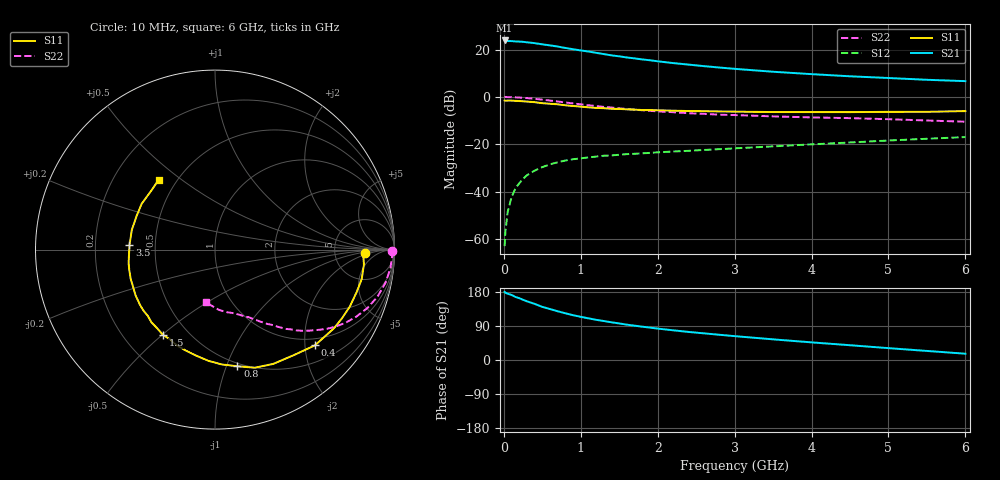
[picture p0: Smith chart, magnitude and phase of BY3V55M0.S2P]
! SIEMENS Small Signal Semiconductors
! BFY420
! Si NPN RF SIEGET Grounded Emitter Transistor in MICRO-X
! VCE = 3.5 V  IC = 5 mA
! Common Emitter S-Parameters:  October  1996
# GHz  S  MA  R  50
!  f  S11  S21  S12  S22
! GHz  MAG  ANG  MAG  ANG  MAG  ANG  MAG  ANG
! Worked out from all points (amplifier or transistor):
!   36 points, 10 MHz to 6 GHz, reference 50 ohm
!   highest |S21| = 23.8 dB at 10 MHz (marker M1)
!   |S21| within 3 dB of that: start of sweep to 771.4 MHz
!   unconditionally stable (mu >= 1): 3.175 GHz to end of sweep
!   at 250 MHz: K = 0.15, MSG = 28.9 dB, |S12| = -34.7 dB
!   at 1.4 GHz: K = 0.53, MSG = 21.1 dB, |S12| = -24.7 dB
!   at 6 GHz: K = 1.13, MAG = 9.6 dB, |S12| = -17.0 dB
!   S11 on the Smith chart (normalised r, x): 10 MHz: 11, -1; 400 MHz: 0.84, -2.22; 800 MHz: 0.47, -1.09; 1.5 GHz: 0.37, -0.50; 3.5 GHz: 0.35, +0.02; 6 GHz: 0.40, +0.41
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0.01  0.8347 -1.3  15.53 179.6  0.0007 57.0  0.988 -0.5
0.02  0.8271 -2.5  15.31 177.6  0.0014 75.2  0.9911 -1.0
0.05  0.8339 -5.7  15.08 174.9  0.0037 76.2  0.9865 -2.7
0.1  0.8337 -11.4  15.06 171.7  0.0076 80.1  0.9834 -5.6
0.15  0.8236 -16.9  14.8 166.5  0.0116 77.8  0.9752 -8.4
0.2  0.8155 -22.9  14.71 163.2  0.0149 76.6  0.9677 -11.0
0.3  0.7951 -33.4  14.2 154.9  0.022 72.6  0.9425 -16.2
0.4  0.7709 -43.8  13.63 148.1  0.0276 66.7  0.9091 -21.0
0.5  0.7337 -53.3  12.85 140.3  0.0327 62.7  0.8721 -25.3
0.6  0.7148 -63.0  12.22 134.5  0.0375 59.3  0.8347 -29.2
0.8  0.662 -79.1  10.78 123.2  0.0451 52.5  0.7601 -35.6
0.9  0.641 -86.6  10.13 118.2  0.0481 50.0  0.7255 -38.1
1.1  0.5996 -100.3  9.053 109.9  0.0526 46.6  0.6646 -42.9
1.3  0.5746 -111.6  7.99 102.8  0.057 43.6  0.6138 -46.4
1.5  0.5564 -121.5  7.173 96.5  0.0597 41.6  0.5717 -49.6
1.8  0.5256 -135.4  6.171 87.9  0.064 39.5  0.5207 -53.4
2.2  0.5107 -150.0  5.165 78.4  0.0699 38.0  0.4737 -57.9
2.8  0.4912 -166.4  4.165 66.6  0.0784 37.2  0.4196 -63.6
3.5  0.4771 177.1  3.389 54.5  0.0899 35.7  0.3863 -69.7
4.5  0.4752 157.1  2.717 39.0  0.1086 32.4  0.3546 -79.4
5.5  0.4828 138.0  2.291 23.9  0.1302 27.3  0.3163 -92.3
6  0.4994 129.0  2.146 16.6  0.1412 24.3  0.2985 -100.0
